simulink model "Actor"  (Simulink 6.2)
settings: Solver=ode45  StartTime=0.0  StopTime=10.0  RelTol=1e-3
undefined symbols (not defined in the file or in its folder): Aa, Ba, Ca, Da

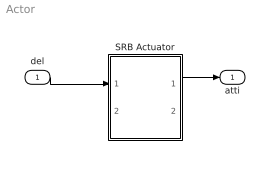
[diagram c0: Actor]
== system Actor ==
  del : Inport  Port=1  LatchInput=off
  SRB Actuator : Subsystem
  atti : Outport
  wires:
  SRB Actuator/1(delto) -> atti/1
  del/1 -> SRB Actuator/1(delti)

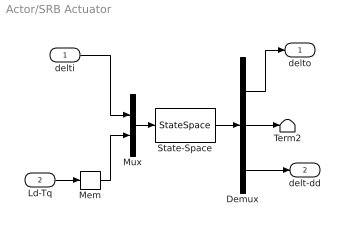
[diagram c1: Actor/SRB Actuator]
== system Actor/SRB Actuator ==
  delti : Inport  Port=1  LatchInput=off
  Ld-Tq : Inport  Port=2  LatchInput=off
  Demux : Demux  Outputs=3
  Mem : Memory
  Mux : Mux  Inputs=2
  State-Space : StateSpace  A=Aa  B=Ba  C=Ca  D=Da
  Term2 : Terminator
  delto : Outport
  delt-dd : Outport  Port=2
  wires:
  Mux/1 -> State-Space/1
  State-Space/1 -> Demux/1
  Demux/1 -> delto/1
  delti/1 -> Mux/1
  Ld-Tq/1 -> Mem/1
  Demux/3 -> delt-dd/1
  Demux/2 -> Term2/1
  Mem/1 -> Mux/2
